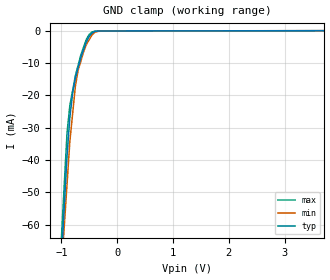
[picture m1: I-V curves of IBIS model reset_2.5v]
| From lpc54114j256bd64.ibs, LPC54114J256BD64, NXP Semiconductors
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[Model] reset_2.5v
Model_type Input
Vinl = 750.000mV
Vinh = 2.00000V
C_comp 1.42000pF 1.40000pF 1.44000pF
[Model spec]
| variable typ   min   max
Vinl  0.750  0.675  0.825
Vinh  2.000  1.800  2.200
| variable typ   min   max
[Voltage Range] 2.50000V 2.25000V 2.75000V
[POWER Clamp Reference] 2.50000V 2.25000V 2.75000V
[GND Clamp Reference] 0.00000V 0.00000V 0.00000V
[Temperature Range]   25   85   -40
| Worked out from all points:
|   GND clamp passes 1 mA (typ) near -0.47 V on its own axis
[GND Clamp]
-2.5V     -547.9mA   -468.9mA   -549.3mA
-900mV    -38.68mA   -47.53mA   -31.64mA
-850mV    -26.92mA   -34.37mA   -23.22mA
-800mV    -19.39mA   -25.73mA   -18.54mA
-750mV    -14.58mA   -17.1mA    -13.85mA
-700mV    -11.35mA   -12.17mA   -10.59mA
-600mV    -5.708mA   -6.37mA    -4.915mA
-550mV    -3.283mA   -4.16mA    -2.496mA
-450mV    -697uA     -1.226mA   -369.5uA
-350mV    -90.67uA   -181.7uA   -104.9uA
-175mV    -57.65uA   -53.91uA   -57.65uA
5V        52.47uA    60.72uA    46.59uA
[POWER Clamp]
-2.5V     0A         0A         0A
5V        0A         0A         0A
